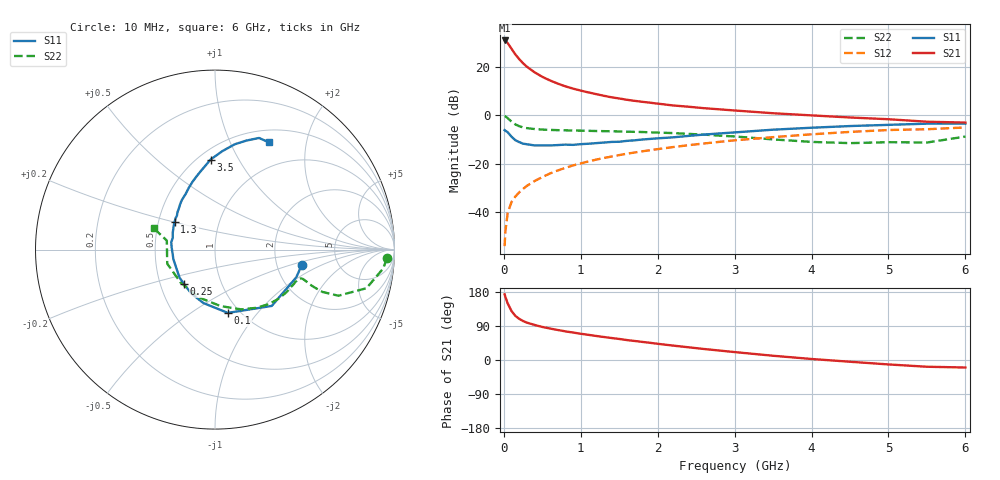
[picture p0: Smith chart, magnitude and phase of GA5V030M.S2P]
! Infineon Technologies  Discrete & RF Semiconductors
! BF775
! Si NPN RF Bipolar Junction Transistor in SOT23
! VCE = 5 V  IC = 30 mA
! Common Emitter S-Parameters:  May  1996
# GHz  S  MA  R  50
!  f  S11  S21  S12  S22
! GHz  MAG  ANG  MAG  ANG  MAG  ANG  MAG  ANG
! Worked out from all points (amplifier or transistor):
!   36 points, 10 MHz to 6 GHz, reference 50 ohm
!   highest |S21| = 30.8 dB at 10 MHz (marker M1)
!   |S21| within 3 dB of that: start of sweep to 90.84 MHz
!   unconditionally stable (mu >= 1): 290.5 MHz to 2.84 GHz
!   at 250 MHz: K = 0.96, MSG = 25.9 dB, |S12| = -30.4 dB
!   at 1.4 GHz: K = 1.14, MAG = 10.0 dB, |S12| = -17.1 dB
!   at 6 GHz: K = 0.95, MSG = 1.0 dB, |S12| = -5.1 dB
!   S11 on the Smith chart (normalised r, x): 10 MHz: 2.78, -0.61; 100 MHz: 0.88, -0.72; 250 MHz: 0.66, -0.27; 1.3 GHz: 0.61, +0.20; 3.5 GHz: 0.57, +0.77; 6 GHz: 0.65, +1.41
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0.01  0.4914 -9.8  34.62 173.2  0.002 88.8  0.959 -2.9
0.02  0.4785 -18.9  33.93 166.5  0.004 84.5  0.943 -6.4
0.05  0.4454 -44.8  30.59 149.3  0.0097 74.0  0.8709 -14.3
0.1  0.3598 -78.5  23.32 129.2  0.0163 66.8  0.734 -20.5
0.15  0.3048 -102.2  17.82 116.3  0.0211 67.0  0.6437 -21.5
0.2  0.2786 -118.0  14.29 108.6  0.0257 68.5  0.5932 -20.8
0.25  0.2587 -131.5  11.73 102.8  0.0303 69.0  0.56 -20.1
0.3  0.2518 -141.8  9.944 98.6  0.035 70.2  0.5405 -19.3
0.4  0.238 -156.3  7.636 92.5  0.044 72.0  0.5183 -18.5
0.5  0.238 -167.1  6.168 87.2  0.053 72.5  0.5045 -18.5
0.6  0.2377 -176.0  5.192 83.1  0.063 73.1  0.4969 -19.0
0.7  0.2422 176.6  4.476 79.2  0.0725 73.1  0.4912 -19.8
0.8  0.2471 170.6  3.929 75.6  0.0822 72.2  0.4875 -20.9
0.9  0.2444 164.5  3.524 72.4  0.0922 72.2  0.4823 -21.9
1.1  0.2581 154.6  2.942 66.4  0.1115 71.1  0.4756 -24.9
1.3  0.2728 145.4  2.51 60.7  0.1314 69.3  0.4685 -27.9
1.6  0.2955 135.0  2.077 52.6  0.1605 66.7  0.4571 -33.2
2.2  0.3494 118.1  1.586 38.0  0.2202 60.9  0.4276 -45.2
3.5  0.5023 92.8  1.096 11.2  0.3528 45.3  0.3167 -84.2
4.5  0.5969 79.4  0.896 -4.6  0.4524 31.3  0.2654 -136.0
5.5  0.6684 68.5  0.733 -17.8  0.5133 15.1  0.2731 169.4
6  0.6692 63.2  0.704 -19.8  0.5585 10.6  0.3626 160.7
